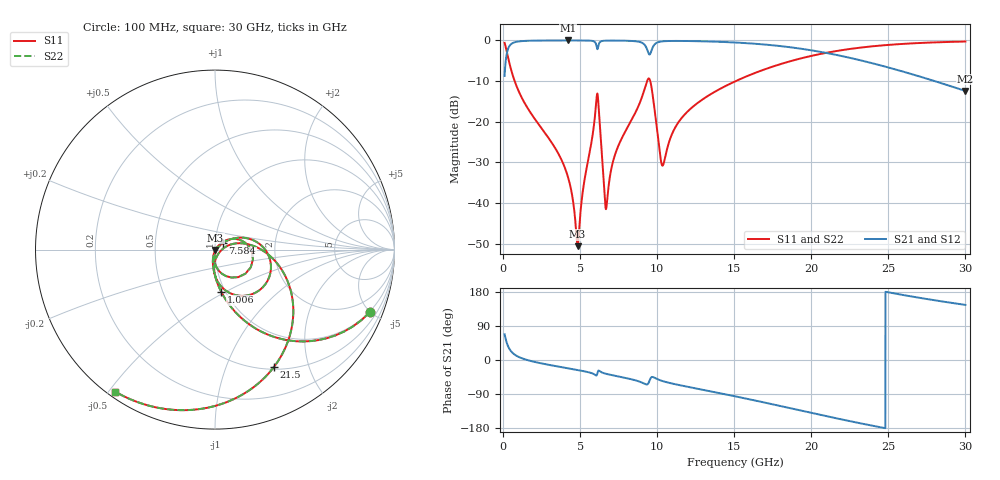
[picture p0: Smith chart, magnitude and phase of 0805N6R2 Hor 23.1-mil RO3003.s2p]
# GHz S MA R 50
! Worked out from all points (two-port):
!   3201 points, 100 MHz to 30 GHz, reference 50 ohm
!   highest |S21| = -0.02 dB at 4.221 GHz (marker M1); lowest = -12.4 dB at 30 GHz (marker M2)
!   |S21| within 3 dB of the highest: 253.5 MHz to 9.421 GHz (9.168 GHz wide, 190 % of centre); 9.582 GHz to 20.88 GHz (11.3 GHz wide, 74.2 % of centre)
!   lowest |S11| = -50.6 dB at 4.837 GHz (marker M3), VSWR 1.01, Z = 50.3 - j0.141 ohm
!   |S11| at or under -10 dB: 751.7 MHz to 9.345 GHz (8.593 GHz wide, 170 % of centre); 9.55 GHz to 15.1 GHz (5.551 GHz wide, 45 % of centre)
!   |S22| runs from -50.6 to -0.3 dB; largest |S21 - S12| = 0
!   S11 on the Smith chart (normalised r, x): 100 MHz: 0.95, -4.97; 1.006 GHz: 0.96, -0.48; 7.584 GHz: 1.09, +0.08; 21.5 GHz: 0.53, -1.49; 30 GHz: 0.02, -0.52
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0.1  0.9305 -22.0  0.3658 68.0  0.3658 68.0  0.9305 -22.0
0.4830937  0.4636 -65.0  0.8854 24.9  0.8854 24.9  0.4636 -65.0
1.006344  0.2389 -81.5  0.97 8.3  0.97 8.3  0.2389 -81.5
4.220594  0.02068 -105.3  0.9972 -22.0  0.9972 -22.0  0.02068 -105.3
4.837281  0.002964 -28.3  0.9969 -26.5  0.9969 -26.5  0.002964 -28.3
5.089563  0.01035 42.4  0.9964 -28.4  0.9964 -28.4  0.01035 42.4
6.070656  0.1991 0.6  0.8414 -40.6  0.8414 -40.6  0.1991 0.6
6.220156  0.1311 -76.6  0.9078 -28.2  0.9078 -28.2  0.1311 -76.6
6.547187  0.01646 -82.4  0.9886 -34.9  0.9886 -34.9  0.01646 -82.4
6.678  0.008437 -25.2  0.9915 -36.4  0.9915 -36.4  0.008437 -25.2
7.584344  0.05621 39.6  0.9921 -44.2  0.9921 -44.2  0.05621 39.6
9.004594  0.199 17.7  0.9366 -59.5  0.9366 -59.5  0.199 17.7
9.434406  0.3397 -28.6  0.6961 -60.9  0.6961 -60.9  0.3397 -28.6
9.668  0.2398 -74.6  0.7844 -44.8  0.7844 -44.8  0.2398 -74.6
10.06978  0.06069 -88.8  0.9507 -51.5  0.9507 -51.5  0.06069 -88.8
10.38747  0.02951 -26.2  0.974 -56.1  0.974 -56.1  0.02951 -26.2
11.72363  0.1193 16.7  0.9828 -68.6  0.9828 -68.6  0.1193 16.7
15.05  0.313 -7.2  0.9414 -95.7  0.9414 -95.7  0.313 -7.2
20.03956  0.6467 -50.6  0.7527 -139.8  0.7527 -139.8  0.6467 -50.6
21.49719  0.7326 -63.5  0.6701 -152.7  0.6701 -152.7  0.7326 -63.5
25.01978  0.8801 -92.2  0.4634 178.4  0.4634 178.4  0.8801 -92.2
30  0.9676 -125.2  0.2389 145.4  0.2389 145.4  0.9676 -125.2
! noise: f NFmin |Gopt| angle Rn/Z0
0.1  0.0007986  0.9229  1.028  0.002293
3.417  0.006316  0.7041  18.97  0.004077
6.743  0.01681  0.7759  36.6  0.01385
10.06  0.0529  0.89  53.62  0.08343
13.39  0.02398  0.716  69.04  0.01147
16.7  0.02826  0.7102  83.38  0.01095
20.03  0.03549  0.7301  96.94  0.01187
23.35  0.0458  0.7619  109.9  0.01335
26.67  0.06102  0.8018  122.6  0.01532
30  0.0848  0.8459  135.3  0.01764
